FUNCTION_BLOCK "IMAC_MOTOR2"
TITLE = MOTOR 2
//--------------------------------------------------------------------------------
//SIEMENS AG     I&S IP PEP SN                      PSP-Element: D-09300081-E-E5
//--------------------------------------------------------------------------------
//History
//=======
//Date      Version  Description                        Author
//1997/06/09   0.6   Basic Edition                      Salge
//2004/06/02   1.0   Converted to S7                    Kahle
//2004/11/05   1.1   Anypointer adjusted                Edelmann
//2004/12/07   1.2   Interface adapted                  Edelmann
//2004/12/07   1.2   Correction feedback-fault          Edelmann
//2004/12/07   1.2   Correction actionfault             Edelmann
//2004/12/07   1.2   Correction change mode             Edelmann
//
//--------------------------------------------------------------------------------
//PLC:   >= S7-300
//--------------------------------------------------------------------------------
//Specification:   Refer "TECHFUNK.DOC"
//--------------------------------------------------------------------------------
//
//--------------------------------------------------------------------------------
//Called FC: FC90 "DELAYTIMER"
//           SFC20 "BLKMOV"
//--------------------------------------------------------------------------------
//
//--------------------------------------------------------------------------------
//Note:
//--------------------------------------------------------------------------------
// KNOW_HOW_PROTECT
AUTHOR : Sa_Ka
FAMILY : IMAC
NAME : Motor2
VERSION : 1.2


VAR_INPUT
  OBJ : INT ;
  RMOT : BOOL ;
  RUN1 : BOOL ;
  RUN2 : BOOL ;
  FAUL : BOOL ;
  ACOM : WORD ;
  BLKO : BOOL ;
  PCONF : STRUCT
   LastRecord : INT  := 100;
   Pointer1stRecord : STRUCT
    S7ID : BYTE  := B#16#10;	//ANY pointer: ID S7
    Typ : BYTE  := B#16#2;	//ANY pointer: data typ =02 BYTE =04 WORD =05 INT =06 DWORD =07 DINT =08 REAL
    RepeatFactor : INT  := 108;	//ANY pointer: repeat factor
    DBNo : INT  := 81;	//ANY pointer: DB number, zero if no DB
    MemoryArea : BYTE  := B#16#84;	//ANY pointer: Memory area =81 IN =82 OUT =83 M =84 DB =85 DI =86 L
    DWHigh : BYTE ;	//ANY pointer: DW highest byte
    DWX : INT ;	//ANY pointer: DW low / bit (address = byte *8 + bit)
   END_STRUCT ;
  END_STRUCT ;
END_VAR
VAR_OUTPUT
  MST1 : BOOL ;
  MST2 : BOOL ;
  MSTO : BOOL ;
  STAT : WORD ;
  OSSTAT : WORD ;	//Status for OS
  OSALARM : WORD ;	//Alarms for OS
END_VAR
VAR_IN_OUT
  OSCOM : WORD ;
END_VAR
VAR
  Motor2 : STRUCT
   System : WORD ;
   CmdOS : WORD ;
   MirrorCmdOS : WORD ;
   Test : WORD ;
   AlarmOS : WORD ;
   StatusOS : WORD ;
   SysStatusOS : WORD ;
   Status1 : WORD ;
   Status2 : WORD ;
   Status3 : BYTE ;
   InputEdges : BYTE ;
   AutoEdges : WORD ;
   DataTimeCmd : STRUCT
    StartTime : DINT ;
    StartEdge : BOOL ;
   END_STRUCT ;
   DataTimeChg12 : STRUCT
    StartTime : DINT ;
    StartEdge : BOOL ;
   END_STRUCT ;
   DataTimeChg21 : STRUCT
    StartTime : DINT ;
    StartEdge : BOOL ;
   END_STRUCT ;
   DataTimeBlackout : STRUCT
    StartTime : DINT ;
    StartEdge : BOOL ;
   END_STRUCT ;
   DataTimeActFault : STRUCT
    StartTime : DINT ;
    StartEdge : BOOL ;
   END_STRUCT ;
   DataTimeExtFault : STRUCT
    StartTime : DINT ;
    StartEdge : BOOL ;
   END_STRUCT ;
   DataTimeFeedback : STRUCT
    StartTime : DINT ;
    StartEdge : BOOL ;
   END_STRUCT ;
   DataTimeAutoAl : STRUCT
    StartTime : DINT ;
    StartEdge : BOOL ;
   END_STRUCT ;
   PCONF : STRUCT
    Modeswitches : STRUCT
     M0_ConstantOut : BOOL ;	// Constant Output MST1 MST2 MSTO (1); Feedback depended Output Anst. (0)
     M1_AutoManLoc : BOOL ;	// AUTO/ MANUAL/ LOCAL (1); MANUAL/ LOCAL (0)
     M2_NoActFeedFault : BOOL ;	// No Action- and Non-Feedback fault(1),
     M3_NoStopIfFault : BOOL ;	// No Stop-Signal if Failure occurs (1)
     M4_RestrtAftBlack : BOOL ;	// Restart after Blackout (1)
     M5_ResetOSonly : BOOL ;	// Reset Alarm only with RESET from OS (1); RESET and START/STOP-Command (0)
     M6_CmdTimeDly : BOOL ;	// Command Time Delay aktiv (1)
     M7_Chg12viaStop : BOOL ;	// Change from 1->2 via STOP(1)
     M8_Chg21viaStop : BOOL ;	// Change from 2->1 via STOP(1)
     M9_StopIfAutoFail : BOOL ;	// NO AVAIL Direct Stop if Auto Failure (1)
     M10_LockBlockCmd : BOOL ;	// Lock blocksCommands
     sw11 : BOOL ;
     sw12 : BOOL ;
     sw13 : BOOL ;
     sw14 : BOOL ;
     sw15 : BOOL ;	//
    END_STRUCT ;
    DlyTCmd : TIME ;	// Setpoint Command time delay
    DlyTBlackout : TIME ;	// Setpoint blackout time delay
    DlyTExtFault : TIME ;	// Setpoint external fault delay
    DlyTFeedback : TIME ;	// Setpoint feedback fault delay
    DlyTActFault : TIME ;	//Setpoint Action Fault delay
    DlyTAutoAl : TIME ;	// Setpoint auto alarm delay
    DlyTRestart : TIME ;	// No AVAIL Setpoint restart after blackout delay
    DlyTChg12 : TIME ;	// Setpoint Waiting Delay 1->2
    DlyTChg21 : TIME ;	// Setpoint Waiting Delay 2->1
   END_STRUCT ;
  END_STRUCT ;
  siFailRR : INT ;	//Failure blockmove read record
  siFailWR : INT ;	//Failure blockmove write record
END_VAR
VAR_TEMP
  tb000 : BOOL ;	//
  tbCmdOSManual : BOOL ;	//    MANUAL
  tbCmdOSAuto : BOOL ;	//    AUTO
  tb003 : BOOL ;	//
  tb004 : BOOL ;	//
  tb005 : BOOL ;	//
  tb006 : BOOL ;	//
  tb007 : BOOL ;	//
  tbCmdOSStart1 : BOOL ;	//    START1 (Manual)
  tbCmdOSStart2 : BOOL ;	//    START2 (Manual)
  tbCmdOSStop : BOOL ;	//    STOP (Manual)
  tb013 : BOOL ;	//
  tb014 : BOOL ;	//
  tb015 : BOOL ;	//
  tb016 : BOOL ;	//
  tbCmdOSReset : BOOL ;	//    RESET
  tbAutoBlackStart1 : BOOL ;	//    Blackoutstart from Auto
  tbAutoBlackStart2 : BOOL ;	//    Blackoutstart2 from Auto
  tb022 : BOOL ;	//
  tb023 : BOOL ;	//
  tb024 : BOOL ;	//
  tb025 : BOOL ;	//
  tb026 : BOOL ;	//
  tbDataReq : BOOL ;	//    Fetch Data requiered
  tb030 : BOOL ;	//
  tb031 : BOOL ;	//
  tbAutoFail : BOOL ;	//    Auto failure input
  tb033 : BOOL ;	//
  tbCmdEmergOff : BOOL ;	//    Command Emergency Off
  tb035 : BOOL ;	//
  tb036 : BOOL ;	//
  tb037 : BOOL ;	//
  tb040 : BOOL ;	//
  tb041 : BOOL ;	//
  tb042 : BOOL ;	//
  tb043 : BOOL ;	//
  tb044 : BOOL ;	//
  tb045 : BOOL ;	//
  tb046 : BOOL ;	//
  tb047 : BOOL ;	//
  tbCmdAutoStart1 : BOOL ;	//    Command Start1 Auto Pulse
  tbCmdAutoStop : BOOL ;	//    Command Stop Auto Pulse
  tbCmdAutoFail : BOOL ;	//    Auto failure input pulse
  tb053 : BOOL ;	//
  tb054 : BOOL ;	//
  tbCmdAutoStart2 : BOOL ;	//    Command Start2 Auto Pulse
  tb056 : BOOL ;	//
  tb057 : BOOL ;	//
  tbRemote : BOOL ;	//    Remote (=1)/ Local
  tbRunning1 : BOOL ;	//    Running1 (=1)/ Stopped
  tbFault : BOOL ;	//    Fault
  tbBlackout : BOOL ;	//    Blackout
  tbRunning2 : BOOL ;	//    Running2 (=1)/ Stopped
  tb065 : BOOL ;	//
  tb066 : BOOL ;	//
  tb067 : BOOL ;	//
  tb070 : BOOL ;	//
  tb071 : BOOL ;	//
  tb072 : BOOL ;	//
  tb073 : BOOL ;	//
  tb074 : BOOL ;	//
  tb075 : BOOL ;	//
  tb076 : BOOL ;	//
  tb077 : BOOL ;	//
  tbStateRun2 : BOOL ;	//    State Running2
  tbStarting2 : BOOL ;	//    State Starting2
  tb082 : BOOL ;	//
  tb083 : BOOL ;	//
  tb084 : BOOL ;	//
  tb085 : BOOL ;	//
  tb086 : BOOL ;	//
  tbSendData : BOOL ;	//    Send Data
  tbStateRun1 : BOOL ;	//    State Running1
  tbStateLocal : BOOL ;	//    State Local
  tbStateManual : BOOL ;	//    State Manual
  tbStateAuto : BOOL ;	//    State Auto
  tbStateFault : BOOL ;	//    State Fault
  tbStateBlackout : BOOL ;	//    State Blackout
  tbStarting1 : BOOL ;	//    State Starting1
  tbReStarting : BOOL ;	//    ReStarting
  tb100 : BOOL ;	//    0: Undefiniert
  tb101 : BOOL ;	//    1: Normal
  tb102 : BOOL ;	//    2: Fault Alarm
  tb103 : BOOL ;	//    3: Auto Alarm
  tb104 : BOOL ;	//    4: Action Alarm
  tb105 : BOOL ;	//    5: Non-Feedback Alarm
  tb106 : BOOL ;	//    6: Locked
  tb107 : BOOL ;	//
  tb110 : BOOL ;	//    7: Emergency Off
  tb111 : BOOL ;	//
  tb112 : BOOL ;	//
  tb113 : BOOL ;	//
  tb114 : BOOL ;	//
  tb115 : BOOL ;	//
  tb116 : BOOL ;	//
  tb117 : BOOL ;	//
  tb120 : BOOL ;	//    0: Undefined
  tb121 : BOOL ;	//    1: RUNNING1 in Local-Mode
  tb122 : BOOL ;	//    2: RUNNING2 in Local-Mode
  tb123 : BOOL ;	//    3: STOPPED in Local-Mode
  tb124 : BOOL ;	//    4: RUNNING1 in Manual-Mode
  tb125 : BOOL ;	//    5: RUNNING2 in Manual-Mode
  tb126 : BOOL ;	//    6: STOPPED in Manual-Mode
  tb127 : BOOL ;	//    7: RUNNING1 in AUTO-Mode
  tb130 : BOOL ;	//    8: RUNNING2 in AUTO-Mode
  tb131 : BOOL ;	//    9: STOPPED in AUTO -Mode
  tb132 : BOOL ;	//    10: WAITING1 in Manual -Mode
  tb133 : BOOL ;	//    11: WAITING2 in Manual -Mode
  tb134 : BOOL ;	//    11: WAITING1 in AUTO-Mode
  tb135 : BOOL ;	//    12: WAITING2 in AUTO-Mode
  tb136 : BOOL ;	//
  tb137 : BOOL ;	//
  tbNonFeedbackTact : BOOL ;	//    Non-Feedback Alarm activ
  tbNonFeedbackA : BOOL ;	//    Non-Feedback Alarm
  tbStartTact : BOOL ;	//    Action Alarm delay activ
  tbActionA : BOOL ;	//    Action Alarm
  tbAutoTact : BOOL ;	//    Autoalarm time delay activ
  tbAutoA : BOOL ;	//    Autoalarm
  tbRun1BeforeBlack : BOOL ;	//    Blackoutstart 1
  tbBlackoutStartTact : BOOL ;	//    Restart time delay activ
  tbStart1 : BOOL ;	//    START1!
  tbStop : BOOL ;	//    STOP!
  tbLocal : BOOL ;	//    LOCAL
  tbManual : BOOL ;	//    MANUAL
  tbAuto : BOOL ;	//    AUTO
  tbCmdTact : BOOL ;	//    Command time delay activ
  tbFaultTact : BOOL ;	//    Fault Input activ
  tbExtFaultA : BOOL ;	//    External Fault alarm
  tb160 : BOOL ;	//
  tb161 : BOOL ;	//
  tb162 : BOOL ;	//
  tbMSTO : BOOL ;	//    Output MSTO
  tbMST1 : BOOL ;	//    Output MST1
  tbMST2 : BOOL ;	//    Output MST2
  tb166 : BOOL ;	//
  tb167 : BOOL ;	//
  tbDlyStop : BOOL ;	//    Delayded Stop
  tbDlyStart1 : BOOL ;	//    Delayded Start1
  tbDlyStart2 : BOOL ;	//    Delayded Start2
  tb173 : BOOL ;	//
  tb174 : BOOL ;	//
  tbStart2 : BOOL ;	//    START2
  tbRun2BeforeBlack : BOOL ;	//    Blackoutstart2
  tb177 : BOOL ;	//
  tbLtRpulse : BOOL ;	//    Local to Remote Pulse
  tb181 : BOOL ;	//
  tb182 : BOOL ;	//
  tb183 : BOOL ;	//
  tb184 : BOOL ;	//
  tb185 : BOOL ;	//
  tb186 : BOOL ;	//
  tb187 : BOOL ;	//
  tbW12Pulse : BOOL ;	//    Wating timer1->2
  tbW21Pulse : BOOL ;	//    Wating timer2->1
  tb192 : BOOL ;	//
  tb193 : BOOL ;	//
  tbStpPulse : BOOL ;	//    Stopping
  tb195 : BOOL ;	//
  tb196 : BOOL ;	//
  tb197 : BOOL ;	//
  tbCmdTexceed : BOOL ;	//    Command Time is over pulse
  tbActTexceed : BOOL ;	//    Action time is over
  tbExtFTexceed : BOOL ;	//    Fault time over
  tbFeedbackTexceed : BOOL ;	//    Non -Feedback time is over
  tbAutoTexceed : BOOL ;	//    Auto failure time is over
  tbReStartTexceed : BOOL ;	//    Restart Time is over
  tbWait12Texecced : BOOL ;	//    waiting time 1->2 is over Pulse
  tbWait21Texecced : BOOL ;	//    waiting time 2->1 is over Pulse
  tbStart1Pulse : BOOL ;	//    START1! Pulse
  tbStopPulse : BOOL ;	//    STOP!Pulse
  tbStart2Pulse : BOOL ;	//    START2! Pulse
  tb213 : BOOL ;	//
  tb214 : BOOL ;	//
  tb215 : BOOL ;	//
  tb216 : BOOL ;	//
  tb217 : BOOL ;	//
  P_currentRecord : ANY ;	//ANY pointer of the current record
END_VAR
BEGIN
NETWORK
TITLE =Calculation of current ANY pointer for reading /writing record
// ANY-pointer of current record
      L     #PCONF.Pointer1stRecord.S7ID;
      T     LB    22;
      L     #PCONF.Pointer1stRecord.Typ;
      T     LB    23;
      L     #PCONF.Pointer1stRecord.RepeatFactor;
      T     LW    24;
      L     #PCONF.Pointer1stRecord.DBNo;
      T     LW    26;
      L     #PCONF.Pointer1stRecord.MemoryArea;
      T     LB    28;
      L     #PCONF.Pointer1stRecord.DWHigh;
      T     LB    29;
      L     #PCONF.Pointer1stRecord.DWX;
      T     LW    30;

      L     #OBJ; //Check whether Obj within the range
      L     #PCONF.LastRecord;
      >I    ;
      SPB   cRcd;
      L     #OBJ;
      L     1;
      <I    ;
      SPB   cRcd;
      L     #OBJ;
cRcd: +     -1;
      L     #PCONF.Pointer1stRecord.RepeatFactor;
      *I    ;
      SLD   3; //DBW + DBX address of the current record
      L     LD    28;
      OD    ;
      T     LD    28; //DBWX part of ANY pointer "P_currentRecord"

NETWORK
TITLE =Read record

      CALL "BLKMOV" (
           SRCBLK                   := #P_currentRecord,
           RET_VAL                  := #siFailRR,
           DSTBLK                   := #Motor2);

NETWORK
TITLE =Read OS command

      L     #OSCOM; // Commands from OS
      T     LW     0;
      L     #Motor2.Status1; // Status stored
      T     LW    14;
      L     #Motor2.Status2; // Status stored
      T     LW    16;
      L     #Motor2.Status3; // Status stored
      T     LB    19;

      L     0; //Reset scratch  flags
      T     LW     6;
      T     LW    20;
      NOP   0;

NETWORK
TITLE = Formaloperanden Inputs

      U     #RMOT;
      =     #tbRemote; // Remote/Local
      U     #RUN1;
      =     #tbRunning1; // Running1
      U     #FAUL;
      =     #tbFault; // Fault
      L     #ACOM;
      T     LW     2; // Command From Automatic
      U     #BLKO;
      =     #tbBlackout; //Blackout
      U     #RUN2;
      =     #tbRunning2; // Running2


// ----Evaluate Pulsflags from Auto Commands----
      L     #Motor2.AutoEdges; //Stored Auto Command last cycle
      INVI  ; //Singlecomplement
      L     LW     2; //Command From Automatic
      T     #Motor2.AutoEdges;
      UW    ;
      T     LW     4; // Command  Pulseflags

// ----Evaluate Pulsflags from Inputs----
      L     #Motor2.InputEdges; //Stored Auto Command last cycle
      INVI  ; //Singlecomplement
      L     LB     6; //Inputs
      T     #Motor2.InputEdges;
      UW    ;
      T     LB    18; // Inputs Pulseflags



//---------------------------------------------------------------------------------

      NOP   0;

NETWORK
TITLE = Local-Manual- Auto

      UN    #tbRemote; // Not Remote
      =     #tbLocal; // LOCAL
      R     #tbManual; // MANUAL!
      R     #tbAuto; // AUTO!
      R     #tbDlyStart1; // DELAYDED START1!
      R     #tbDlyStart2; // DELAYDED START2!
      R     #tbDlyStop; // DELAYDED STOP!
      R     #tbCmdTact; // reset COMMAND TIMER ACTIV
      R     #tbStart1; // START1!
      R     #tbStart2; // START2!
      R     #tbStop; // STOP!
      R     #tbRun1BeforeBlack; // BLACKOUT START 1
      R     #tbRun2BeforeBlack; // BLACKOUT START 2
      R     #tbNonFeedbackTact; // reset Non Feedback Timer
      R     #tbStartTact; // reset Action Timer
      R     #tbAutoTact; // reset Auto Timer
      R     #tbW12Pulse; // reset Wating timer1->2
      R     #tbW21Pulse; // reset Wating timer2->1
      R     #tbStpPulse; // reset Stopping


      SPB   NE03;
      U     #Motor2.PCONF.Modeswitches.M1_AutoManLoc; // extra Automode ?
      SPB   MODE;
      S     #tbManual; //MANUAL!
      S     #tbAuto; // AUTO!
      SPA   NE03;
MODE: U     #tbCmdOSManual; //Command Manual
      S     #tbManual; //MANUAL!
      R     #tbAuto; // AUTO!
      U     #tbCmdOSAuto; //Command Auto
      S     #tbAuto; // AUTO!
      R     #tbManual; // MANUAL!
      UN    #tbAuto; // AUTO!
      UN    #tbManual; // MANUAL!
      S     #tbManual; // MANUAL!
NE03: NOP   0;

NETWORK
TITLE = Commands
//-------SET Start 1 Command----------
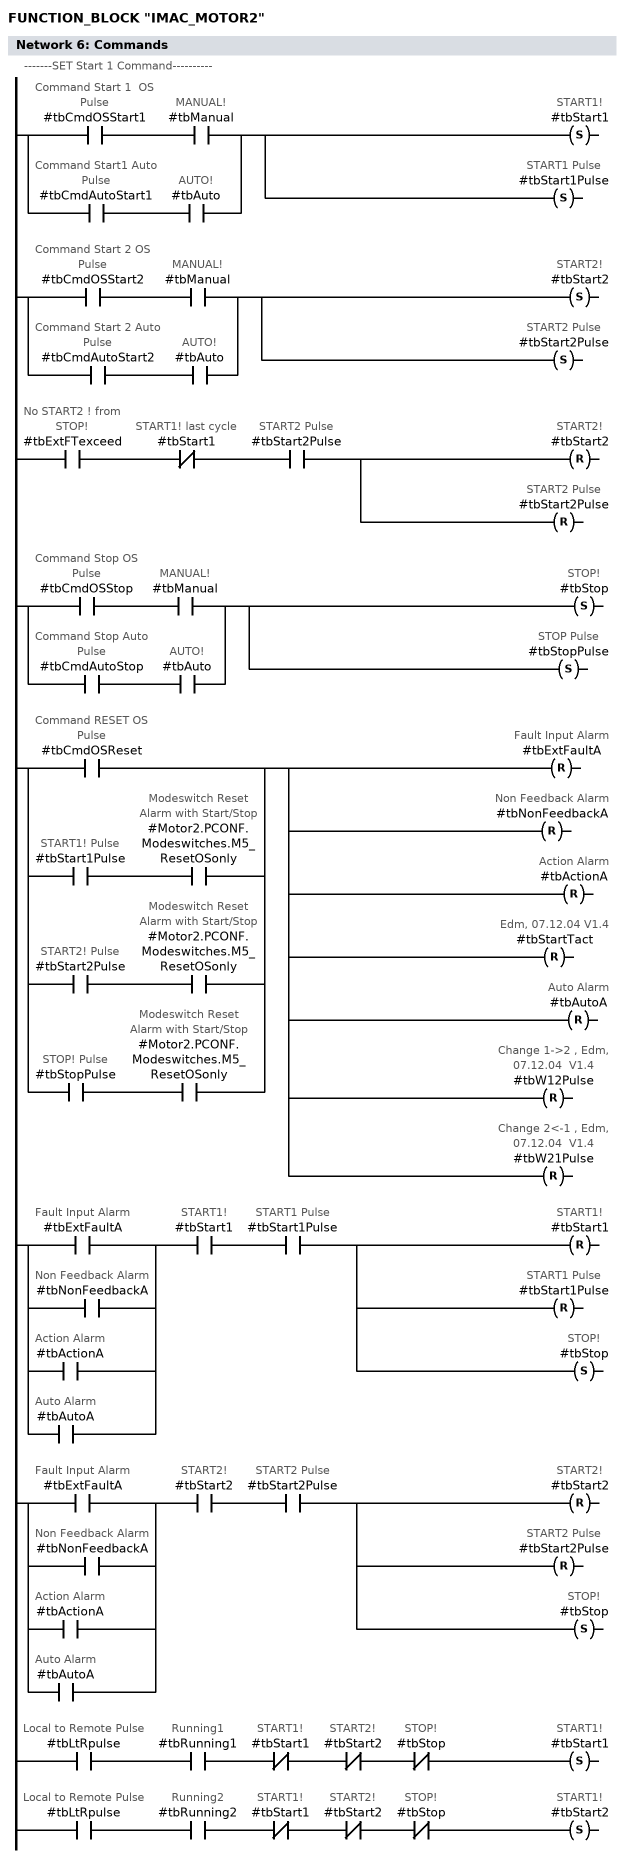
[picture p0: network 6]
      O(    ;
      U     #tbCmdOSStart1; //Command Start 1  OS Pulse
      U     #tbManual; // MANUAL!
      )     ;
      O(    ;
      U     #tbCmdAutoStart1; //Command Start1 Auto Pulse
      U     #tbAuto; // AUTO!
      )     ;
      S     #tbStart1; // START1!
      S     #tbStart1Pulse; // START1 Pulse

//-------SET Start 2 Command----------

      O(    ;
      U     #tbCmdOSStart2; //Command Start 2 OS Pulse
      U     #tbManual; // MANUAL!
      )     ;
      O(    ;
      U     #tbCmdAutoStart2; //Command Start 2 Auto Pulse
      U     #tbAuto; // AUTO!
      )     ;
      S     #tbStart2; // START2!
      S     #tbStart2Pulse; // START2 Pulse

      U     #tbExtFTexceed; // No START2 ! from STOP!
      UN    #tbStart1; // START1! last cycle
      U     #tbStart2Pulse; // START2 Pulse
      R     #tbStart2; // START2!
      R     #tbStart2Pulse; // START2 Pulse

//-------SET Stop Command----------
      O(    ;
      U     #tbCmdOSStop; //Command Stop OS Pulse
      U     #tbManual; // MANUAL!
      )     ;
      O(    ;
      U     #tbCmdAutoStop; //Command Stop Auto Pulse
      U     #tbAuto; // AUTO!
      )     ;
      S     #tbStop; // STOP!
      S     #tbStopPulse; // STOP Pulse

//-------Reset Alarms----------
      O     #tbCmdOSReset; //Command RESET OS Pulse
      O(    ;
      U     #tbStart1Pulse; // START1! Pulse
      U     #Motor2.PCONF.Modeswitches.M5_ResetOSonly; // Modeswitch Reset Alarm with Start/Stop
      )     ;
      O(    ;
      U     #tbStart2Pulse; // START2! Pulse
      U     #Motor2.PCONF.Modeswitches.M5_ResetOSonly; // Modeswitch Reset Alarm with Start/Stop
      )     ;
      O(    ;
      U     #tbStopPulse; // STOP! Pulse
      U     #Motor2.PCONF.Modeswitches.M5_ResetOSonly; // Modeswitch Reset Alarm with Start/Stop
      )     ;
      R     #tbExtFaultA; // Fault Input Alarm
      R     #tbNonFeedbackA; // Non Feedback Alarm
      R     #tbActionA; // Action Alarm
      R     #tbStartTact; // Edm, 07.12.04 V1.4
      R     #tbAutoA; // Auto Alarm
      R     #tbW12Pulse; //Change 1->2 , Edm, 07.12.04  V1.4
      R     #tbW21Pulse; //Change 2<-1 , Edm, 07.12.04  V1.4

//-------Reset START ! if Failure----------
      O     #tbExtFaultA; // Fault Input Alarm
      O     #tbNonFeedbackA; // Non Feedback Alarm
      O     #tbActionA; // Action Alarm
      O     #tbAutoA; // Auto Alarm
      U     #tbStart1; // START1!
      U     #tbStart1Pulse; // START1 Pulse
      R     #tbStart1; // START1!
      R     #tbStart1Pulse; // START1 Pulse
      S     #tbStop; // STOP!


      O     #tbExtFaultA; // Fault Input Alarm
      O     #tbNonFeedbackA; // Non Feedback Alarm
      O     #tbActionA; // Action Alarm
      O     #tbAutoA; // Auto Alarm
      U     #tbStart2; // START2!
      U     #tbStart2Pulse; // START2 Pulse
      R     #tbStart2; // START2!
      R     #tbStart2Pulse; // START2 Pulse
      S     #tbStop; // STOP!

//-------Local Remote change ----------
      U     #tbLtRpulse; // Local to Remote Pulse
      U     #tbRunning1; // Running1
      UN    #tbStart1; // START1!
      UN    #tbStart2; // START2!
      UN    #tbStop; // STOP!
      S     #tbStart1; // START1!

      U     #tbLtRpulse; // Local to Remote Pulse
      U     #tbRunning2; // Running2
      UN    #tbStart1; // START1!
      UN    #tbStart2; // START2!
      UN    #tbStop; // STOP!
      S     #tbStart2; // START1!

      NOP   0;


NETWORK
TITLE = Command Time Delay

      UN    #Motor2.PCONF.Modeswitches.M6_CmdTimeDly; // no Modeswitch Command time delay ?
      SPB   NE05;
      U     #tbCmdTact; // COMMAND TIMER ACTIV
      U     #tbStart1Pulse; // START1! Pulse
      R     #tbStart1Pulse; // reset START1! Pulse
      R     #tbStart1; // reset START!
      S     #tbDlyStart1; // DELAYDED START1!
      R     #tbDlyStart2; // DELAYDED START2!
      R     #tbDlyStop; // DELAYDED STOP!

      U     #tbCmdTact; // COMMAND TIMER ACTIV
      U     #tbStart2Pulse; // START2! Pulse
      R     #tbStart2Pulse; // reset START2! Pulse
      R     #tbStart2; // reset START2!
      S     #tbDlyStart2; // DELAYDED START2!
      R     #tbDlyStart1; // DELAYDED START1!
      R     #tbDlyStop; // DELAYDED STOP!


      U     #tbCmdTact; // COMMAND TIMER ACTIV
      U     #tbStopPulse; // STOP! Pulse
      R     #tbStopPulse; // reset STOP! Pulse
      R     #tbStop; // reset STOP!
      S     #tbDlyStop; // DELAYDED STOP!
      R     #tbDlyStart1; // DELAYDED START1!
      R     #tbDlyStart2; // DELAYDED START1!

      O     #tbStart1Pulse; // START1! Pulse
      O     #tbStart2Pulse; // START2! Pulse
      O     #tbStopPulse; // STOP! Pulse
      S     #tbCmdTact; // set COMMAND TIMER ACTIV

      CALL "IMAC_DELAYTIMER" (
           XSTART                   := #tbCmdTact,
           XTIME                    := #Motor2.PCONF.DlyTCmd,
           YON                      := #tbCmdTexceed,
           MEM                      := #Motor2.DataTimeCmd);

      U     #tbCmdTexceed; // Command Time is over pulse
      U     #tbDlyStart1; // DELAYDED START1!
      S     #tbStart1; // START1!
      S     #tbStart1Pulse; // START1! Pulse
      R     #tbDlyStop; // DELAYDED START!

      U     #tbCmdTexceed; // Command Time is over pulse
      U     #tbDlyStart2; // DELAYDED START2!
      S     #tbStart2; // START2!
      S     #tbStart2Pulse; // START2! Pulse
      R     #tbDlyStart2; // DELAYDED START2!
      U     #tbCmdTexceed; // Command Time is over pulse
      U     #tbDlyStop; // DELAYDED STOP!
      S     #tbStop; // STOP!
      S     #tbStopPulse; // STOP! Pulse
      R     #tbDlyStop; // DELAYDED STOP!
NE05: NOP   0;

NETWORK
TITLE = Change Mode
//--- STOP von 1nach 0 ----//
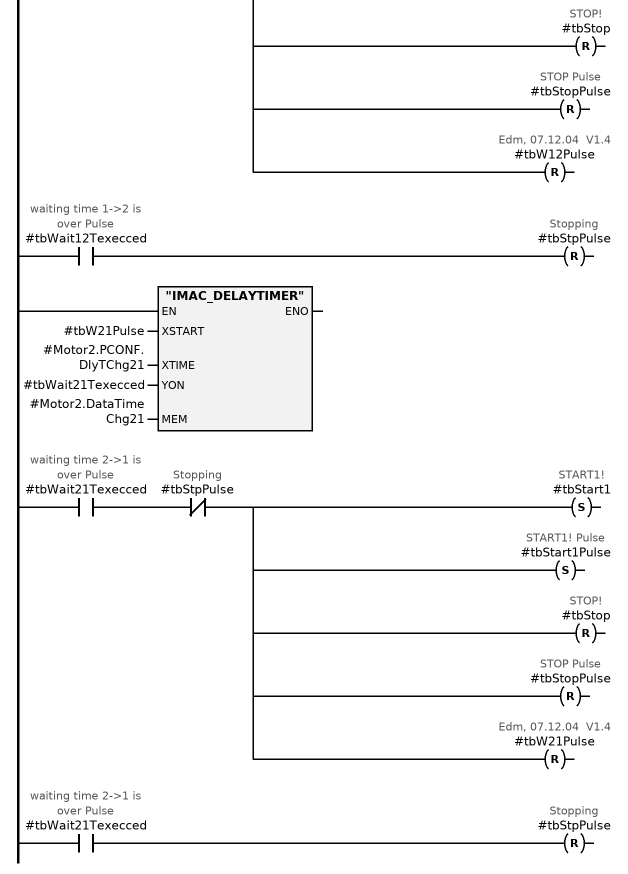
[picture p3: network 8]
      U     #tbStart1; // START1!
      U     #tbStopPulse; // STOP Pulse
      R     #tbW21Pulse; // Waiting time 2->1 activ
//      S     #tbW12Pulse                 // Waiting time 1->2 activ  Edm,07.12.04
      S     #tbStpPulse; // Stopping !

//--- STOP von 2 nach 0----//
      U     #tbStart2; // START2!
      U     #tbStopPulse; // STOP Pulse
//      S     #tbW21Pulse                 // Waiting time 2->1 activ  Edm,07.12.04
      R     #tbW12Pulse; // Waiting time 1->2 activ
      S     #tbStpPulse; // Stopping !
//Stopping wenn Stop Befehl
      O     #tbW21Pulse; // Waiting time 2->1 activ
      O     #tbW12Pulse; // Waiting time 1->2 activ
      U     #tbStopPulse; // STOP Pulse
      UN    #tbStpPulse; // Stopping
      S     #tbStpPulse; // Stopping !


//--- Wechsel von 1 nach 2----//
      U     #tbStart1; // START1! last cycle
      U     #tbStart2Pulse; // START2! Pulse
      U     #Motor2.PCONF.Modeswitches.M7_Chg12viaStop; // MOD Change from 1->2 via Stop
      S     #tbStop; // STOP!
      S     #tbStopPulse; // STOP Pulse

      U     #tbStart1; // START1! last cycle
      U     #tbStart2Pulse; // START2! Pulse
      R     #tbW21Pulse; // Waiting time 2->1 activ
      R     #tbStpPulse; // Stopping
      R     #tbStart2; // START2!
      R     #tbStart2Pulse; // START2! Pulse
      R     #tbStart1; // START1! last cycle
      S     #tbW12Pulse; // Waiting time 1->2 activ

//--- Wechsel von 2 nach 1----//
      U     #tbStart2; // START2! last cycle
      U     #tbStart1Pulse; // START1! Pulse
      U     #Motor2.PCONF.Modeswitches.M8_Chg21viaStop; // MOD Change from 2->1 via Stop
      S     #tbStop; // STOP!
      S     #tbStopPulse; // STOP Pulse


      U     #tbStart2; // START2! last cycle
      U     #tbStart1Pulse; // START1! Pulse
      R     #tbW12Pulse; // Waiting time 1->2 activ
      R     #tbStpPulse; // Stopping
      R     #tbStart1; // START1!
      R     #tbStart1Pulse; // START1! Pulse
      R     #tbStart2; // START2! last cycle
      S     #tbW21Pulse; // Waiting time 2->1 activ



//----Wechsel STOP nach 1-------
//Rüchsetze Stopping wenn neuer Start befehl kommt---//:
      U     #tbStart1Pulse; // START1! Pulse
      U     #tbW21Pulse; // Waiting time 2->1 activ
      R     #tbStpPulse; // Stopping
      R     #tbStart1; // START1!
      R     #tbStart1Pulse; // START1! Pulse

//Rücksetze stopping und falsche  Wating time wenn alter Befehl wieder kommt
      U     #tbStart1Pulse; // START1! Pulse
      U     #tbW12Pulse; // Waiting time 1->2 activ
      R     #tbStpPulse; // Stopping
      R     #tbW12Pulse; // Waiting time 1->2 activ

//----Wechsel STOP nach 2-------
//Rüchsetze Stopping wenn neuer Start befehl kommt---//:
      U     #tbStart2Pulse; // START2! Pulse
      U     #tbW12Pulse; // Waiting time 1->2 activ
      R     #tbStpPulse; // Stopping
      R     #tbStart2; // START2!
      R     #tbStart2Pulse; // START2! Pulse

//Rücksetze Stopping und falsche Wating time wenn alter Befehl wieder kommt
      U     #tbStart2Pulse; // START2! Pulse
      U     #tbW21Pulse; // Waiting time 2->1 activ
      R     #tbStpPulse; // Stopping
      R     #tbW21Pulse; // Waiting time 2->1 activ

//----Waiting Timer 1->2
      CALL "IMAC_DELAYTIMER" (
           XSTART                   := #tbW12Pulse,
           XTIME                    := #Motor2.PCONF.DlyTChg12,
           YON                      := #tbWait12Texecced,
           MEM                      := #Motor2.DataTimeChg12);

      U     #tbWait12Texecced; //waiting time 1->2 is over Pulse
      UN    #tbStpPulse; // Stopping
      S     #tbStart2; // START2!
      S     #tbStart2Pulse; // START2! Pulse
      R     #tbStop; // STOP!
      R     #tbStopPulse; // STOP Pulse
      R     #tbW12Pulse; //Edm, 07.12.04  V1.4

      U     #tbWait12Texecced; //waiting time 1->2 is over Pulse
      R     #tbStpPulse; // Stopping

//----Waiting Timer 2->1
      CALL "IMAC_DELAYTIMER" (
           XSTART                   := #tbW21Pulse,
           XTIME                    := #Motor2.PCONF.DlyTChg21,
           YON                      := #tbWait21Texecced,
           MEM                      := #Motor2.DataTimeChg21);

      U     #tbWait21Texecced; //waiting time 2->1 is over Pulse
      UN    #tbStpPulse; // Stopping
      S     #tbStart1; // START1!
      S     #tbStart1Pulse; // START1! Pulse
      R     #tbStop; // STOP!
      R     #tbStopPulse; // STOP Pulse
      R     #tbW21Pulse; //Edm, 07.12.04  V1.4

      U     #tbWait21Texecced; //waiting time 2->1 is over Pulse
      R     #tbStpPulse; // Stopping

      NOP   0;

NETWORK
TITLE = Restart after Blackout
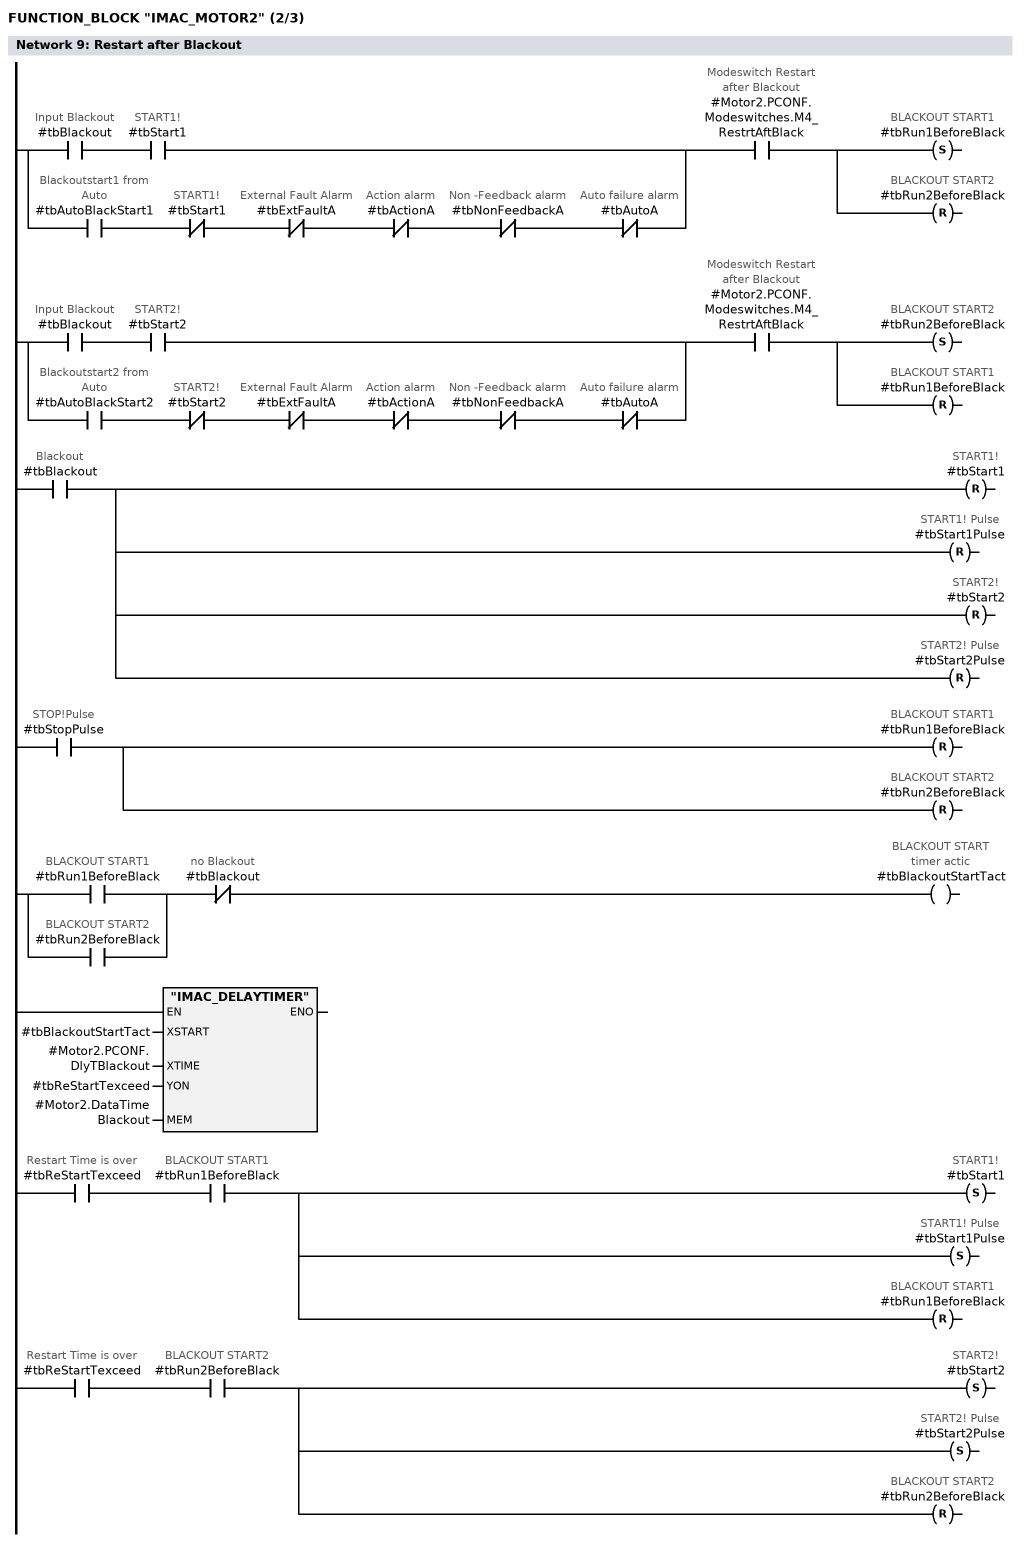
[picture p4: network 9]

      O(    ;
      U     #tbBlackout; // Input Blackout
      U     #tbStart1; // START1!
      )     ;
      O(    ;
      U     #tbAutoBlackStart1; // Blackoutstart1 from  Auto
      UN    #tbStart1; // START1!
      UN    #tbExtFaultA; // External Fault Alarm
      UN    #tbActionA; // Action alarm
      UN    #tbNonFeedbackA; // Non -Feedback alarm
      UN    #tbAutoA; // Auto failure alarm
      )     ;
      U     #Motor2.PCONF.Modeswitches.M4_RestrtAftBlack; // Modeswitch Restart after Blackout
      S     #tbRun1BeforeBlack; // BLACKOUT START1
      R     #tbRun2BeforeBlack; // BLACKOUT START2

      O(    ;
      U     #tbBlackout; // Input Blackout
      U     #tbStart2; // START2!
      )     ;
      O(    ;
      U     #tbAutoBlackStart2; // Blackoutstart2 from  Auto
      UN    #tbStart2; // START2!
      UN    #tbExtFaultA; // External Fault Alarm
      UN    #tbActionA; // Action alarm
      UN    #tbNonFeedbackA; // Non -Feedback alarm
      UN    #tbAutoA; // Auto failure alarm
      )     ;
      U     #Motor2.PCONF.Modeswitches.M4_RestrtAftBlack; // Modeswitch Restart after Blackout
      S     #tbRun2BeforeBlack; // BLACKOUT START2
      R     #tbRun1BeforeBlack; // BLACKOUT START1

      U     #tbBlackout; // Blackout
      R     #tbStart1; // START1!
      R     #tbStart1Pulse; // START1! Pulse
      R     #tbStart2; // START2!
      R     #tbStart2Pulse; // START2! Pulse

      U     #tbStopPulse; // STOP!Pulse
      R     #tbRun1BeforeBlack; // BLACKOUT START1
      R     #tbRun2BeforeBlack; // BLACKOUT START2

      O     #tbRun1BeforeBlack; // BLACKOUT START1
      O     #tbRun2BeforeBlack; // BLACKOUT START2
      UN    #tbBlackout; //  no Blackout
      =     #tbBlackoutStartTact; // BLACKOUT START timer actic
      CALL "IMAC_DELAYTIMER" (
           XSTART                   := #tbBlackoutStartTact,
           XTIME                    := #Motor2.PCONF.DlyTBlackout,
           YON                      := #tbReStartTexceed,
           MEM                      := #Motor2.DataTimeBlackout);
      U     #tbReStartTexceed; // Restart Time is over
      U     #tbRun1BeforeBlack; // BLACKOUT START1
      S     #tbStart1; // START1!
      S     #tbStart1Pulse; // START1! Pulse
      R     #tbRun1BeforeBlack; // BLACKOUT START1

      U     #tbReStartTexceed; // Restart Time is over
      U     #tbRun2BeforeBlack; // BLACKOUT START2
      S     #tbStart2; // START2!
      S     #tbStart2Pulse; // START2! Pulse
      R     #tbRun2BeforeBlack; // BLACKOUT START2

      NOP   0;

NETWORK
TITLE = Reset old states
// -----Rücksetzen des alten Status-----(Sonst in NW Commands)------
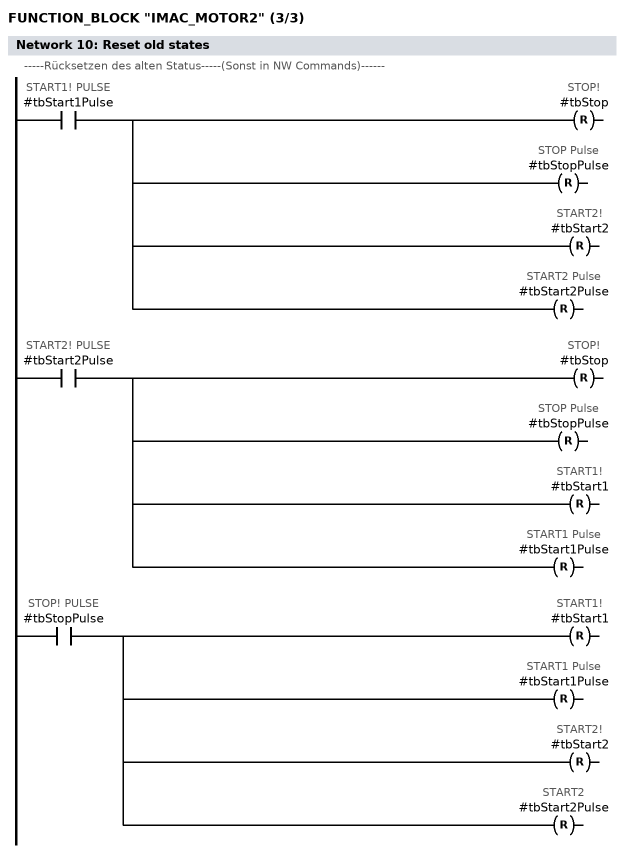
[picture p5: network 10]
      U     #tbStart1Pulse; // START1! PULSE
      R     #tbStop; // STOP!
      R     #tbStopPulse; // STOP Pulse
      R     #tbStart2; // START2!
      R     #tbStart2Pulse; // START2 Pulse

      U     #tbStart2Pulse; // START2! PULSE
      R     #tbStop; // STOP!
      R     #tbStopPulse; // STOP Pulse
      R     #tbStart1; // START1!
      R     #tbStart1Pulse; // START1 Pulse

      U     #tbStopPulse; // STOP! PULSE
      R     #tbStart1; // START1!
      R     #tbStart1Pulse; // START1 Pulse
      R     #tbStart2; // START2!
      R     #tbStart2Pulse; // START2

      NOP   0;

NETWORK
TITLE = Action Alarm

      U     #Motor2.PCONF.Modeswitches.M2_NoActFeedFault; // No Action and Feedback alarm
      SPB   NE07;
      O     #tbStart1Pulse; // START1! Pulse
      O     #tbStart2Pulse; // START2! Pulse
      S     #tbStartTact; // Action Timer activ

      CALL "IMAC_DELAYTIMER" (
           XSTART                   := #tbStartTact,
           XTIME                    := #Motor2.PCONF.DlyTActFault,
           YON                      := #tbActTexceed,
           MEM                      := #Motor2.DataTimeActFault);

      U     #tbActTexceed; // Action time is over
      S     #tbActionA; // Action alarm
      U     #tbActTexceed; // Action time is over
      UN    #Motor2.PCONF.Modeswitches.M3_NoStopIfFault; // Modswitch  Stop iif alarm
      R     #tbStart1; // START1!
      R     #tbStart1Pulse; // START1! Pulse
      R     #tbStart2; // START2!
      R     #tbStart2Pulse; // START2! Pulse
      S     #tbStop; // STOP!
      S     #tbStopPulse; // STOP! Pulse

      O(    ;
      U     #tbRunning1; // Running 1
      U     #tbStart1; // START1
      )     ;
      O(    ;
      U     #tbRunning2; // Running 2
      U     #tbStart2; // START2!
      )     ;
      O     #tbStop; // STOP!
      O     #tbBlackout; // Blackout
      R     #tbStartTact; // reset Action Timer

NE07: NOP   0;

NETWORK
TITLE = External Fault Alarm

      O     #tbAuto; // AUTO!
      O     #tbManual; // MANUAL!
      SPB   RMOT;
      U     #tbFault; // External Fault
      =     #tbExtFaultA; // External Fault Alarm
      SPA   NE08;
RMOT: U     #tbFault; // External Fault
      UN    #tbExtFaultA; // External Fault Alarm
      UN    #tbBlackout; // Blackout
      =     #tbFaultTact; // Fault timer activ

      CALL "IMAC_DELAYTIMER" (// Timer External Fault
           XSTART                   := #tbFaultTact,
           XTIME                    := #Motor2.PCONF.DlyTExtFault,
           YON                      := #tbExtFTexceed,
           MEM                      := #Motor2.DataTimeExtFault);

      U     #tbExtFTexceed; // Fault time over
      S     #tbExtFaultA; // External Fault Alarm
      R     #tbStart1; // START1!
      R     #tbStart1Pulse; // START1! Pulse
      R     #tbStart2; // START2!
      R     #tbStart2Pulse; // START2! Pulse
      S     #tbStop; // STOP!
      S     #tbStopPulse; // STOP! Pulse

NE08: NOP   0;

NETWORK
TITLE = Non-Feedback alarm

      U     #Motor2.PCONF.Modeswitches.M2_NoActFeedFault; // Modeswitch No Action and Feedback alarm
      SPB   NE09;
      O     #tbStart1; // START1!
      O     #tbStart2; // START2!
      UN    #tbRunning1; // not Running1
      UN    #tbRunning2; // not Running2
      UN    #tbStartTact; // no Action Timer activ
      UN    #tbActionA; // no Action alarm
      UN    #tbFaultTact; // no Fault timer activ
      UN    #tbExtFaultA; // no External Fault Alarm
      UN    #tbBlackout; // no Blackout
      =     #tbNonFeedbackTact; // Non -Feedback Timer activ

      CALL "IMAC_DELAYTIMER" (// Timer Non Feedback alarm delay
           XSTART                   := #tbNonFeedbackTact,
           XTIME                    := #Motor2.PCONF.DlyTFeedback,
           YON                      := #tbFeedbackTexceed,
           MEM                      := #Motor2.DataTimeFeedback);//Edm, 07.12.04 V1.3

      U     #tbFeedbackTexceed; // Non -Feedback time is over
      S     #tbNonFeedbackA; // Non -Feedback alarm
      U     #tbFeedbackTexceed; // Non -Feedback time is over
      UN    #Motor2.PCONF.Modeswitches.M3_NoStopIfFault; // Modswitch  Stop iif alarm
      R     #tbStart1; // START1!
      R     #tbStart1Pulse; // START1! Pulse
      R     #tbStart2; // START2!
      R     #tbStart2Pulse; // START2! Pulse
      S     #tbStop; // STOP!
      S     #tbStopPulse; // STOP! Pulse

NE09: NOP   0;

NETWORK
TITLE = Auto Failure

      UN    #tbAuto; // not in AUTO! Mode
      SPB   NE10;
      U     #tbCmdAutoFail; // Auto failure Input pulse
      S     #tbAutoTact; // Auto failure Timer activ
      UN    #tbAutoFail; // Auto failure Input
      R     #tbAutoTact; // Auto failure Timer activ

      CALL "IMAC_DELAYTIMER" (
           XSTART                   := #tbAutoTact,
           XTIME                    := #Motor2.PCONF.DlyTAutoAl,
           YON                      := #tbAutoTexceed,
           MEM                      := #Motor2.DataTimeAutoAl);

      U     #tbAutoTexceed; // Auto failure time is over
      S     #tbAutoA; // Auto failure alarm
      U     #tbAutoTexceed; // Auto failure time is over
      U     #tbActTexceed; // Modeswitch Delayded AutoFault with Stop
      R     #tbStart1; // START1!
      R     #tbStart1Pulse; // START1! Pulse
      R     #tbStart2; // START2!
      R     #tbStart2Pulse; // START2! Pulse
      S     #tbStop; // STOP!
      S     #tbStopPulse; // STOP! Pulse


NE10: NOP   0;

NETWORK
TITLE = Automatic States
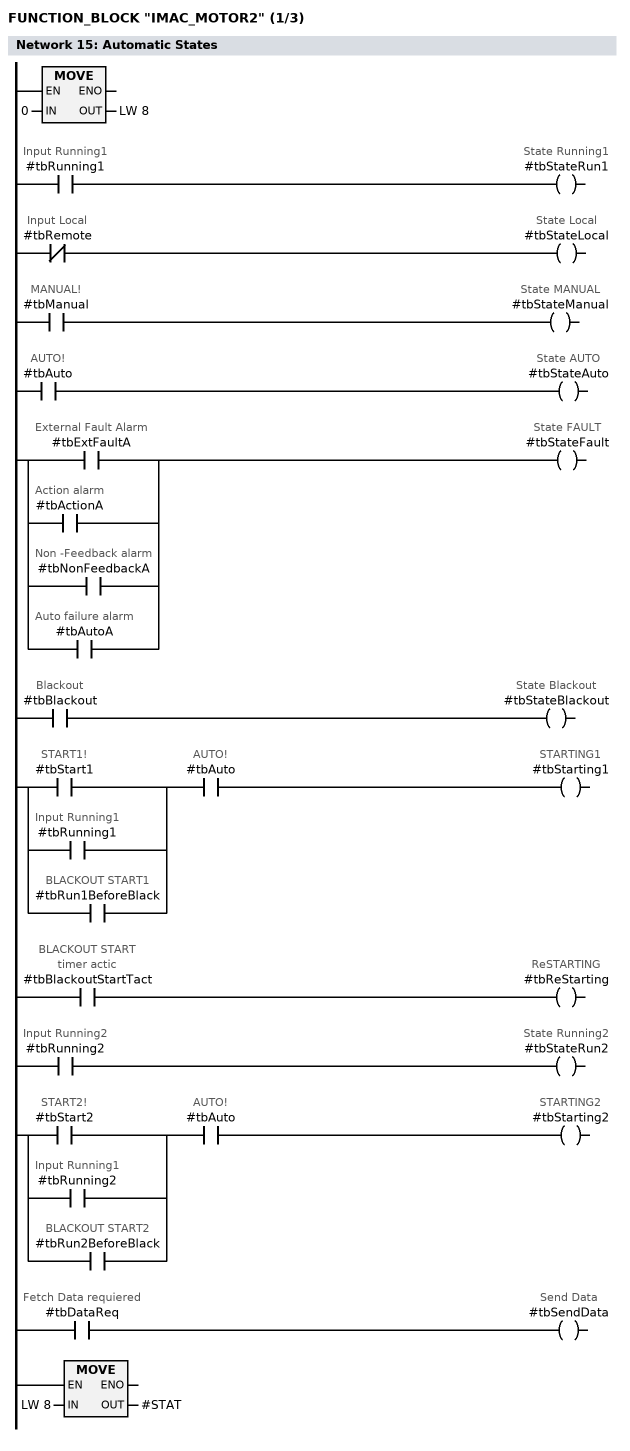
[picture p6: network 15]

      L     0;
      T     LW     8;
      U     #tbRunning1; // Input Running1
      =     #tbStateRun1; // State Running1
      UN    #tbRemote; // Input Local
      =     #tbStateLocal; // State Local
      U     #tbManual; // MANUAL!
      =     #tbStateManual; // State MANUAL
      U     #tbAuto; // AUTO!
      =     #tbStateAuto; // State AUTO
      O     #tbExtFaultA; // External Fault Alarm
      O     #tbActionA; // Action alarm
      O     #tbNonFeedbackA; // Non -Feedback alarm
      O     #tbAutoA; // Auto failure alarm
      =     #tbStateFault; // State FAULT
      U     #tbBlackout; // Blackout
      =     #tbStateBlackout; // State Blackout
      O     #tbStart1; // START1!
      O     #tbRunning1; // Input Running1
      O     #tbRun1BeforeBlack; // BLACKOUT START1
      U     #tbAuto; // AUTO!
      =     #tbStarting1; // STARTING1
      U     #tbBlackoutStartTact; // BLACKOUT START timer actic
      =     #tbReStarting; // ReSTARTING
      U     #tbRunning2; // Input Running2
      =     #tbStateRun2; // State Running2
      O     #tbStart2; // START2!
      O     #tbRunning2; // Input Running1
      O     #tbRun2BeforeBlack; // BLACKOUT START2
      U     #tbAuto; // AUTO!
      =     #tbStarting2; // STARTING2
      U     #tbDataReq; // Fetch Data requiered
      =     #tbSendData; // Send Data

      L     LW     8; // State To Automatic
      T     #STAT;

      NOP   0;

NETWORK
TITLE = Lock/ Emergency Off
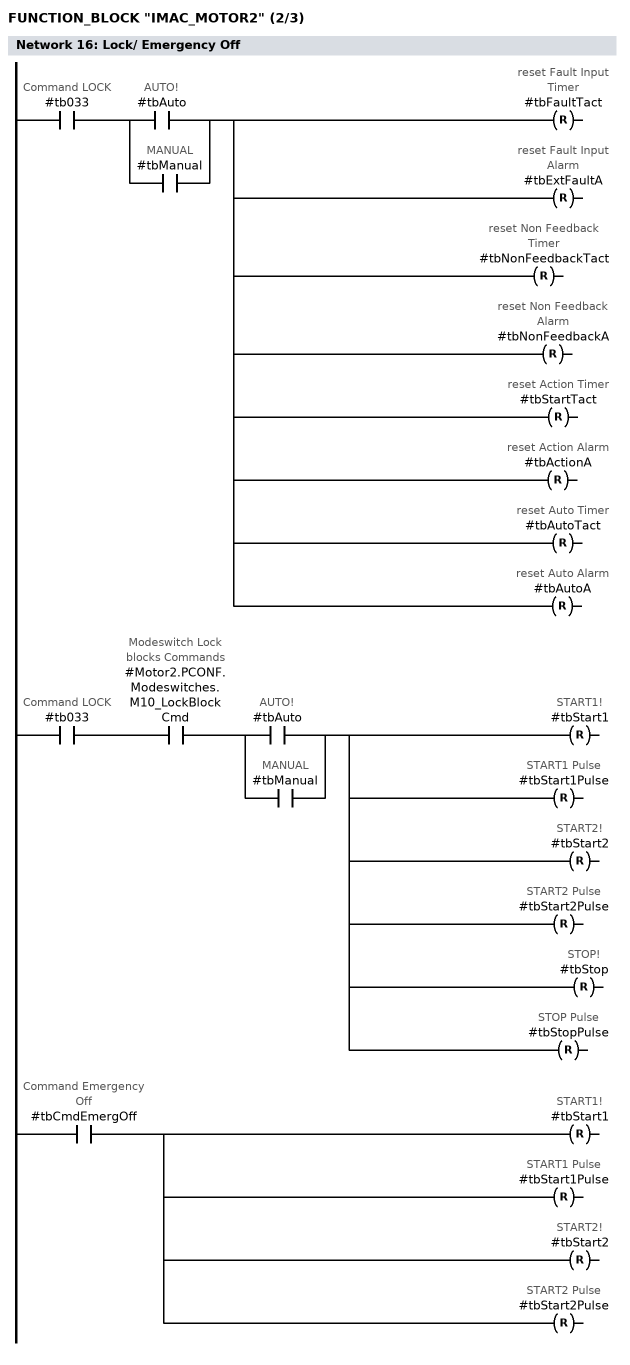
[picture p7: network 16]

      U     #tb033; //Command LOCK
      U(    ;
      O     #tbAuto; // AUTO!
      O     #tbManual; // MANUAL
      )     ;
      R     #tbFaultTact; // reset Fault Input Timer
      R     #tbExtFaultA; // reset Fault Input Alarm
      R     #tbNonFeedbackTact; // reset Non Feedback Timer
      R     #tbNonFeedbackA; // reset Non Feedback Alarm
      R     #tbStartTact; // reset Action Timer
      R     #tbActionA; // reset Action Alarm
      R     #tbAutoTact; // reset Auto Timer
      R     #tbAutoA; // reset Auto Alarm

      U     #tb033; //Command LOCK
      U     #Motor2.PCONF.Modeswitches.M10_LockBlockCmd; //Modeswitch Lock blocks Commands
      U(    ;
      O     #tbAuto; // AUTO!
      O     #tbManual; // MANUAL
      )     ;
      R     #tbStart1; // START1!
      R     #tbStart1Pulse; // START1 Pulse
      R     #tbStart2; // START2!
      R     #tbStart2Pulse; // START2 Pulse
      R     #tbStop; // STOP!
      R     #tbStopPulse; // STOP Pulse

//----Emergency Off
      U     #tbCmdEmergOff; //Command Emergency Off
      R     #tbStart1; // START1!
      R     #tbStart1Pulse; // START1 Pulse
      R     #tbStart2; // START2!
      R     #tbStart2Pulse; // START2 Pulse


      NOP   0;


NETWORK
TITLE = Output
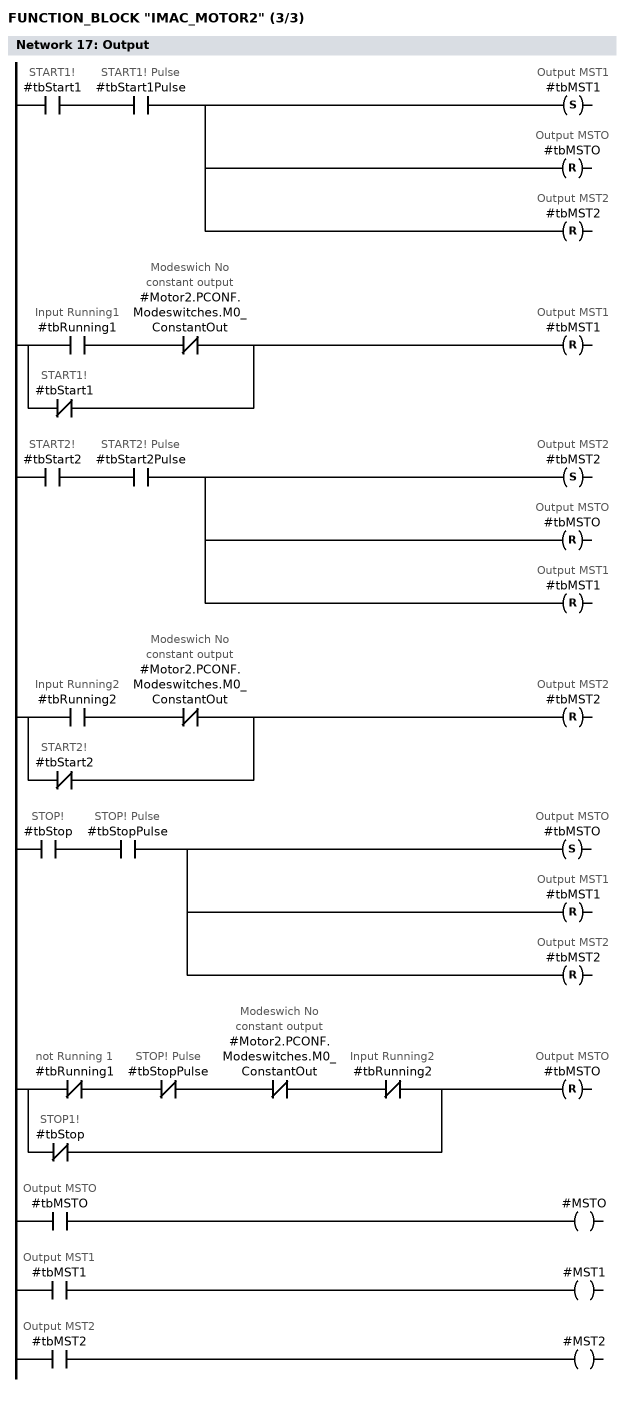
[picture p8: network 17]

      U     #tbStart1; // START1!
      U     #tbStart1Pulse; // START1! Pulse
      S     #tbMST1; // Output MST1
      R     #tbMSTO; // Output MSTO
      R     #tbMST2; // Output MST2
      U     #tbRunning1; // Input Running1
      UN    #Motor2.PCONF.Modeswitches.M0_ConstantOut; // Modeswich No constant output
      ON    #tbStart1; // START1!
      R     #tbMST1; // Output MST1

      U     #tbStart2; // START2!
      U     #tbStart2Pulse; // START2! Pulse
      S     #tbMST2; // Output MST2
      R     #tbMSTO; // Output MSTO
      R     #tbMST1; // Output MST1
      U     #tbRunning2; // Input Running2
      UN    #Motor2.PCONF.Modeswitches.M0_ConstantOut; // Modeswich No constant output
      ON    #tbStart2; // START2!
      R     #tbMST2; // Output MST2

      U     #tbStop; // STOP!
      U     #tbStopPulse; // STOP! Pulse
      S     #tbMSTO; // Output MSTO
      R     #tbMST1; // Output MST1
      R     #tbMST2; // Output MST2

      UN    #tbRunning1; // not Running 1
      UN    #tbStopPulse; // STOP! Pulse
      UN    #Motor2.PCONF.Modeswitches.M0_ConstantOut; // Modeswich No constant output
      UN    #tbRunning2; // Input Running2
      ON    #tbStop; // STOP1!
      R     #tbMSTO; // Output MSTO

      U     #tbMSTO; // Output MSTO
      =     #MSTO;
      U     #tbMST1; // Output MST1
      =     #MST1;
      U     #tbMST2; // Output MST2
      =     #MST2;

      NOP   0;

NETWORK
TITLE = Combinate States
//----Alarms----
      U     #tb033; //Command LOCK
      U(    ;
      O     #tbAuto; // AUTO!
      O     #tbManual; // MANUAL
      )     ;
      L     6; // Lock
      SPB   COD1;
      U     #tbCmdEmergOff; // Emergency Off
      L     7;
      SPB   COD1;

      UN    #tbExtFaultA; // External Fault Alarm
      UN    #tbActionA; // Action alarm
      UN    #tbNonFeedbackA; // Non -Feedback alarm
      UN    #tbAutoA; // Auto failure alarm
      UN    #tbBlackout; // Input Blackout
      L     1; // Normal
      SPB   COD1;
      U     #tbExtFaultA; // External Fault Alarm
      L     2;
      SPB   COD1;
      U     #tbAutoA; // Auto failure alarm
      L     3;
      SPB   COD1;
      U     #tbActionA; // Action alarm
      L     4;
      SPB   COD1;
      U     #tbNonFeedbackA; // Non -Feedback alarm
      L     5;
      SPB   COD1;
      U     #tbBlackout; // Input Blackout
      L     8;
      SPB   COD1;

      L     0; //Undefined
COD1: T     LW    10; //States to OS

//----Status----

      O     #BLKO; //Backout
      O     #tbBlackoutStartTact; // BLACKOUT START timer actic
      L     7; //Blackout
      SPB   COD2;
      U     #tbRunning1; //Input Running1
      L     1; //Running1
      SPB   COD2;
      U     #tbRunning2; //Input Running2
      L     2; //Running2
      SPB   COD2;
//     U     #tbAuto; // AUTO!
//     UN    #tbStartTact; // START Timer activ
//     UN    #tbExtFaultA; // External Fault Alarm
//     UN    #tbActionA; // Action alarm
//     UN    #tbNonFeedbackA; // Non -Feedback alarm
//     UN    #tbAutoA; // Auto failure alarm
//     UN    #tbBlackout; // Input Blackout
//     U     #tbAutoStbyCtrl; //Standbycontrol active
//     L     6; //Standby
//     SPB   COD2;
      UN    #tbRunning1; //Not Running1
      U     #tbMST1; // START1!
      L     4; //Starting1
      SPB   COD2;
      UN    #tbRunning2; //Not Running2
      U     #tbMST2; // START2!
      L     5; //Starting2
      SPB   COD2;
      UN    #tbRunning1; //Running1
      UN    #tbRunning2; //Running2
      L     3; //Stopped
      SPB   COD2;
      L     0; //Undefined
COD2: T     LW    12; //States to OS

      UN    #tbRemote; //Local?
      L     256;
      SPB   COD3;
      U     #tbManual; //Manual?
      L     512;
      SPB   COD3;
      U     #tbAuto; // AUTO?
      L     1024;
      SPB   COD3;
      L     0;
COD3: L     LW    12; //Basic states
      +I    ;
      T     LW    12; //Combinate states to OS

NETWORK
TITLE = Store States in Record

      L     0; // Reset Commands OS
      T     #Motor2.CmdOS;
      T     #OSCOM; // Write Reset Back to I/O interface  added: 20060619 /Ho
      L     LW    10;
      T     #Motor2.AlarmOS; // Alarms to OS
      T     #OSALARM;
      L     LW    12;
      T     #Motor2.StatusOS; // States to OS
      T     #OSSTAT;
      L     LW    14;
      T     #Motor2.Status1; // Status stored
      L     LW    16;
      T     #Motor2.Status2; // Status stored
      L     LB    19;
      T     #Motor2.Status3; // Status stored

NETWORK
TITLE =Write record

      CALL "BLKMOV" (
           SRCBLK                   := #Motor2,
           RET_VAL                  := #siFailWR,
           DSTBLK                   := #P_currentRecord);


END_FUNCTION_BLOCK

